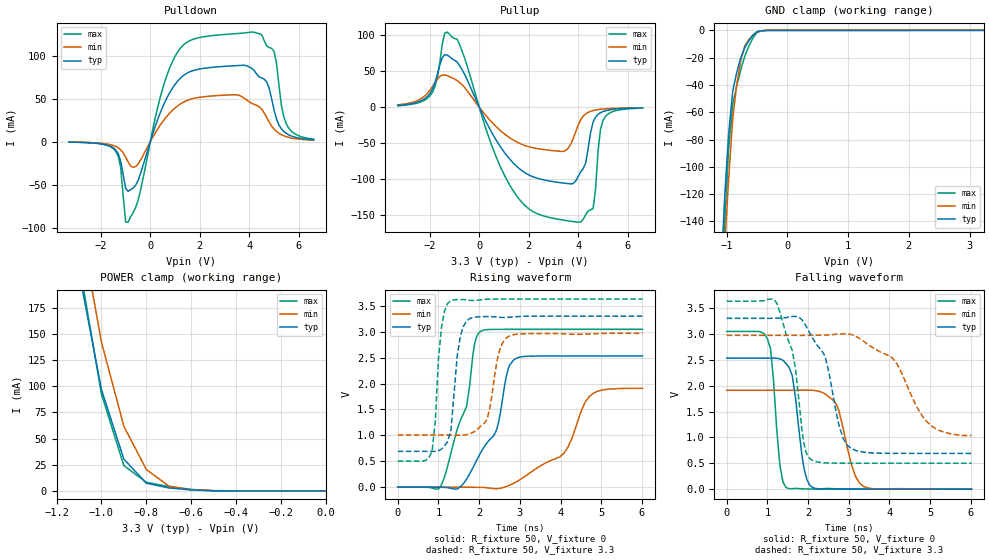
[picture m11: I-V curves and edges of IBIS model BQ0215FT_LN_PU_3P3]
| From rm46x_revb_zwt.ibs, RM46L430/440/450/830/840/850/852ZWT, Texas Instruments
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|   Model Cell BQ0215FT_LN_PU_3P3
|BQ0215FT_LN_PU_3P3
[Model]   BQ0215FT_LN_PU_3P3
Model_type   I/O
Polarity   Non-Inverting
Enable   Active-Low
Vinl =  1.15
Vinh =  1.55
Cref =  15.0001pF
Rref =  101.0000M
Vref =  0V
Vmeas =  1.65
C_comp   1.2p   1.2p   1.2p
[Model Spec]
Vinl   1.15   1.02   1.28
Vinh   1.55   1.45   1.65
[Temperature Range]   25   155   -40
[Voltage Range]   3.3   2.97   3.63
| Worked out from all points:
|   slope of the pulldown table from 0 to 0.495 V, typ, clamps not added: 12.4 ohm
|   slope of the pullup table from 0 to 0.495 V, typ, clamps not added: 14.3 ohm
|   GND clamp passes 1 mA (typ) near -0.50 V on its own axis
|   POWER clamp passes 1 mA (typ) near -0.60 V on its own axis
|   rising waveform, R_fixture 50, V_fixture 0: 20-80 % time 710ps typ, 1.09ns min, 539ps max; typ from 0 V to 2.53 V
|   rising waveform, R_fixture 50, V_fixture 3.3: 20-80 % time 191ps typ, 255ps min, 163ps max; typ from 0.691 V to 3.3 V
|   falling waveform, R_fixture 50, V_fixture 0: 20-80 % time 236ps typ, 354ps min, 181ps max; typ from 2.53 V to 0 V
|   falling waveform, R_fixture 50, V_fixture 3.3: 20-80 % time 544ps typ, 833ps min, 396ps max; typ from 3.3 V to 0.691 V
[POWER_clamp]
|   voltage   I(typ)   I(min)   I(max)
-3.3V     3.99A      4.579A     4.788A
-1.1V     209.6mA    262.2mA    219.1mA
-1.067V   172.1mA    222.3mA    177mA
-1.033V   134.5mA    182.3mA    134.9mA
-1V       96.98mA    142.4mA    92.77mA
-900mV    30.42mA    61.81mA    24.22mA
-800mV    7.461mA    20.58mA    8.236mA
-700mV    2.845mA    4.596mA    4.214mA
-600mV    944uA      1.092mA    1.45mA
-500mV    147.5uA    237.2uA    206.1uA
0V        545.1pA    11.95nA    507.5pA
[Pulldown]
|   voltage   I(typ)   I(min)   I(max)
-3.3V     -654.8uA   -577.8uA   -653.2uA
-1.4V     -9.819mA   -5.703mA   -11.25mA
-1V       -54.51mA   -18.05mA   -93.7mA
-900mV    -57.81mA   -23.76mA   -93.76mA
-500mV    -45.49mA   -26.36mA   -68.8mA
500mV     40.37mA    23.25mA    61.83mA
1.1V      70.16mA    41.36mA    104mA
4.1V      85.11mA    44.32mA    127.2mA
4.7V      69.58mA    28.18mA    111.1mA
5V        36.79mA    14.44mA    104.9mA
5.5V      9.351mA    5.597mA    20.3mA
6.6V      2.027mA    1.639mA    2.825mA
[Pullup]
|   voltage   I(typ)   I(min)   I(max)
-3.3V     2.63mA     3.499mA    2.212mA
-1.9V     24.96mA    28.62mA    20.66mA
-1.3V     72.58mA    44.01mA    104.4mA
-800mV    58.09mA    34.42mA    87.13mA
500mV     -34.83mA   -20.49mA   -52.76mA
1.4V      -78.18mA   -45.94mA   -117.3mA
3.4V      -105.1mA   -61.11mA   -156.5mA
4V        -95.77mA   -24.34mA   -159.4mA
4.3V      -77.12mA   -9.018mA   -149mA
4.6V      -20.57mA   -4.498mA   -140.3mA
5V        -5.887mA   -2.35mA    -18.3mA
6.6V      -811.7uA   -570.8uA   -1.147mA
[GND_clamp]
|   voltage   I(typ)   I(min)   I(max)
-3.3V     -3.262A    -2.882A    -4.97A
-1.1V     -186.6mA   -218.5mA   -219.6mA
-1.033V   -123.2mA   -160.3mA   -142.3mA
-966.7mV  -75.95mA   -109.1mA   -87.16mA
-900mV    -44.75mA   -64.89mA   -54.33mA
-833.3mV  -30.85mA   -39.93mA   -40.7mA
-766.7mV  -20.13mA   -22.06mA   -28.89mA
-700mV    -12.58mA   -11.27mA   -18.91mA
-566.7mV  -3.669mA   -3.357mA   -5.646mA
-500mV    -992.9uA   -1.176mA   -1.493mA
-300mV    -23.36uA   -20.8uA    -38.78uA
3.233V    -1.26uA    5.635uA    -10.55uA
[Ramp]
| variable   typ   min   max
dV/dt_f   1.588147/0.5667661n   1.196794/0.8994973n   1.902872/0.4074894n
dV/dt_r   1.543913/0.7280839n   1.16467/1.136421n   1.858316/0.5494469n
R_load = 50
[Rising Waveform]
R_fixture = 50
V_fixture = 0
V_fixture_min = 0
V_fixture_max = 0
|   time   V(typ)   V(min)   V(max)
0s        188.1uV    151.3uV    215.7uV
1.076ns   -3.087mV   144.5uV    49.13mV
1.692ns   153.9mV    -1.034mV   1.559V
1.888ns   438.9mV    -2.79mV    2.764V
2.028ns   651.3mV    -3.761mV   3.002V
2.436ns   1.124V     -30.37mV   3.045V
2.86ns    2.464V     78.86mV    3.046V
4.084ns   2.531V     655mV      3.046V
4.8ns     2.531V     1.809V     3.046V
6.016ns   2.531V     1.908V     3.046V
[Rising Waveform]
R_fixture = 50
V_fixture = 3.3
V_fixture_min = 2.97
V_fixture_max = 3.63
|   time   V(typ)   V(min)   V(max)
0s        691mV      1.006V     501.8mV
844ps     689.8mV    1.006V     685.2mV
1.076ns   733.8mV    1.006V     3.087V
1.308ns   1.102V     1.006V     3.601V
1.536ns   2.903V     1.004V     3.621V
1.768ns   3.254V     1.029V     3.606V
2.208ns   3.292V     1.347V     3.628V
2.484ns   3.281V     2.592V     3.63V
2.712ns   3.278V     2.906V     3.63V
6.016ns   3.3V       2.97V      3.63V
[Falling Waveform]
R_fixture = 50
V_fixture = 0
V_fixture_min = 0
V_fixture_max = 0
|   time   V(typ)   V(min)   V(max)
0s        2.531V     1.91V      3.046V
1ns       2.531V     1.91V      2.906V
1.076ns   2.532V     1.91V      2.716V
1.308ns   2.516V     1.91V      460.3mV
1.46ns    2.424V     1.91V      31.36mV
1.612ns   2.188V     1.91V      9.196mV
2.072ns   55.18mV    1.911V     3.017mV
2.712ns   6.842mV    1.611V     398.4uV
3.368ns   1.072mV    50.02mV    243.9uV
6.016ns   201.9uV    838.5uV    215.7uV
[Falling Waveform]
R_fixture = 50
V_fixture = 3.3
V_fixture_min = 2.97
V_fixture_max = 3.63
|   time   V(typ)   V(min)   V(max)
0s        3.3V       2.97V      3.63V
1.228ns   3.303V     2.97V      3.599V
1.612ns   3.336V     2.97V      2.678V
1.888ns   3.231V     2.97V      928.2mV
2.072ns   2.972V     2.971V     573.5mV
2.392ns   2.604V     2.976V     509.8mV
3.064ns   783.9mV    2.987V     502.2mV
4.084ns   691.8mV    2.526V     501.8mV
5ns       691mV      1.244V     501.7mV
6.016ns   691mV      1.036V     501.7mV
